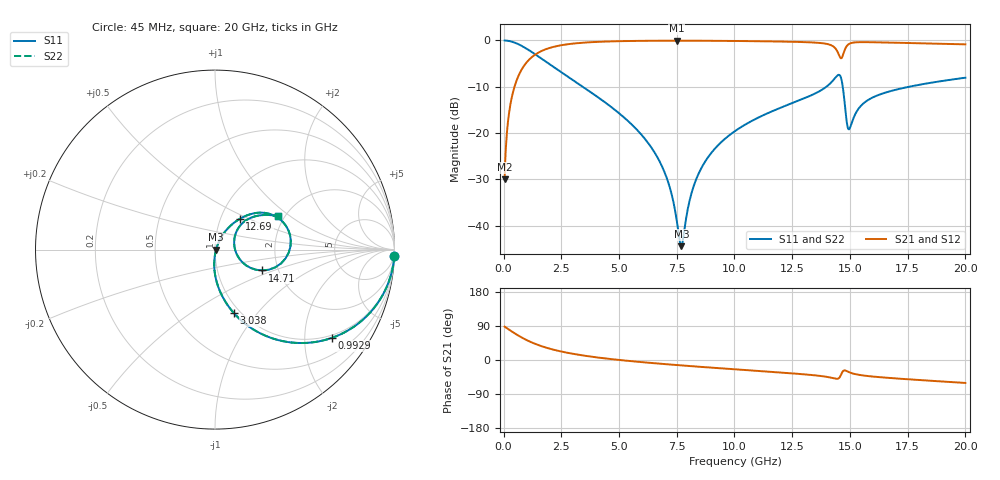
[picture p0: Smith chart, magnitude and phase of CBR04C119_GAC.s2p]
! S-parameter model data by Modelithics Inc.  support@modelithics.com 813-866-6335  Tampa FL USA
! S-Parameter data specifications:
! Substrate: 20-mil Rogers 4350B, substrate thickness, H=0.508mm, Dielectric constant, Er=3.75
! PCB Mounting Pad Footprint: Pad width, PadW=0.52mm , Pad length, PadL=0.52mm , Pad gap, PadG (edge-to-edge)=0.28mm , Reference planes=1.32mm apart
#  GHz  S  MA  R 50
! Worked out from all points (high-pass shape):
!   801 points, 45 MHz to 20 GHz, reference 50 ohm
!   highest |S21| = -0.05 dB at 7.503 GHz (marker M1); lowest = -30.0 dB at 45 MHz (marker M2)
!   |S21| within 3 dB of the highest: 1.37 GHz to 14.52 GHz (13.15 GHz wide, 166 % of centre); 14.7 GHz to end of sweep
!   lowest |S11| = -44.4 dB at 7.703 GHz (marker M3), VSWR 1.01, Z = 50.6 - j0.106 ohm
!   |S11| at or under -10 dB: 3.432 GHz to 13.98 GHz (10.54 GHz wide, 121 % of centre); 14.69 GHz to 17.56 GHz (2.866 GHz wide, 17.8 % of centre)
!   |S22| runs from -44.4 to 0.0 dB; largest |S21 - S12| = 0
!   S11 on the Smith chart (normalised r, x): 45 MHz: 1, -60; 992.9 MHz: 0.92, -2.70; 3.038 GHz: 0.93, -0.76; 12.69 GHz: 1.23, +0.44; 14.71 GHz: 1.65, -0.42; 20 GHz: 1.84, +0.81
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0.045  0.9995 -1.9  0.0316 88.1  0.0316 88.1  0.9995 -1.9
0.219606  0.9883 -9.2  0.1526 80.8  0.1526 80.8  0.9883 -9.2
0.369269  0.9677 -15.3  0.2516 74.7  0.2516 74.7  0.9677 -15.3
0.992862  0.8152 -37.2  0.5779 52.8  0.5779 52.8  0.8152 -37.2
1.915781  0.5715 -58.5  0.8181 31.3  0.8181 31.3  0.5715 -58.5
3.03825  0.3683 -73.5  0.9262 16.0  0.9262 16.0  0.3683 -73.5
3.387462  0.3217 -76.9  0.943 12.5  0.943 12.5  0.3217 -76.9
6.704981  0.05244 -93.4  0.9929 -9.4  0.9929 -9.4  0.05244 -93.4
7.178913  0.02695 -89.4  0.9937 -11.8  0.9937 -11.8  0.02695 -89.4
7.503181  0.01124 -71.6  0.9938 -13.4  0.9938 -13.4  0.01124 -71.6
7.702731  0.006031 -10.0  0.9937 -14.3  0.9937 -14.3  0.006031 -10.0
8.500931  0.03904 62.6  0.9926 -18.0  0.9926 -18.0  0.03904 62.6
10.0225  0.1052 61.5  0.987 -24.6  0.987 -24.6  0.1052 61.5
12.69148  0.2201 51.1  0.9649 -36.2  0.9649 -36.2  0.2201 51.1
13.36496  0.2586 47.2  0.9518 -39.7  0.9518 -39.7  0.2586 47.2
14.28788  0.3748 31.0  0.8582 -48.1  0.8582 -48.1  0.3748 31.0
14.53732  0.4252 6.6  0.6868 -47.0  0.6868 -47.0  0.4252 6.6
14.71193  0.2876 -23.9  0.7126 -28.6  0.7126 -28.6  0.2876 -23.9
14.98631  0.1119 17.3  0.9239 -32.7  0.9239 -32.7  0.1119 17.3
15.56001  0.2068 43.9  0.9588 -40.7  0.9588 -40.7  0.2068 43.9
16.68248  0.2805 40.5  0.9483 -47.2  0.9483 -47.2  0.2805 40.5
20  0.3963 28.0  0.9073 -60.5  0.9073 -60.5  0.3963 28.0
